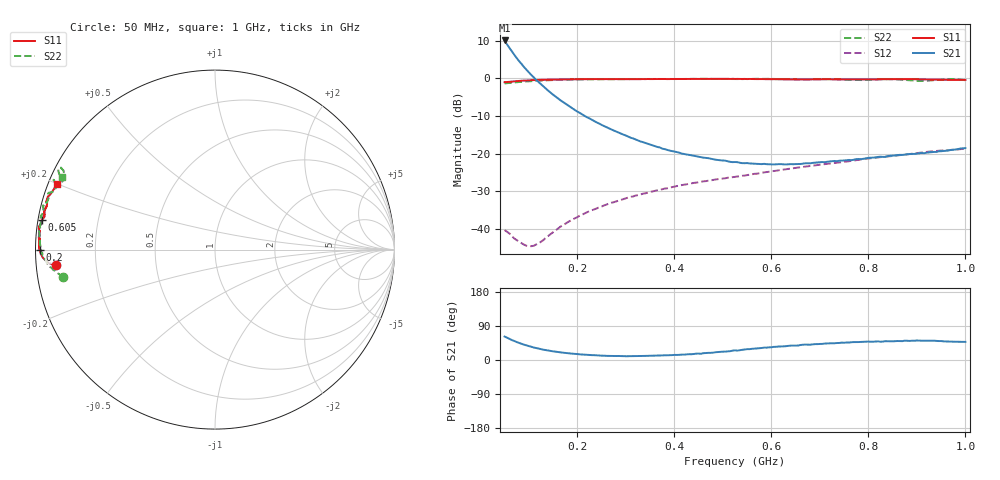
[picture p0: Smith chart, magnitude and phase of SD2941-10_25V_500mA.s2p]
!Agilent Technologies,E8358A,US42080673,A.04.86
!Agilent E8358A: A.04.86
!Date: Friday, June 09, 2006 14:44:03
!Correction: S11(Full 2 Port SOLT,1,2) S21(Full 2 Port SOLT,1,2) S12(Full 2 Port SOLT,1,2) S22(Full 2 Port SOLT,1,2)
!S2P File: Measurements: S11, S21, S12, S22:
# Hz S  MA  R 50
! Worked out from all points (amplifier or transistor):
!   191 points, 50 MHz to 1 GHz, reference 50 ohm
!   highest |S21| = 10.1 dB at 50 MHz (marker M1)
!   |S21| within 3 dB of that: start of sweep to 65.27 MHz
!   unconditionally stable (mu >= 1): 638.1 MHz to 683.3 MHz; 731.3 MHz to 825.9 MHz; 861.3 MHz to 965.3 MHz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
!   at 205 MHz: K = 0.28, MSG = 13.6 dB, |S12| = -36.4 dB
!   at 525 MHz: K = 0.64, MSG = 2.0 dB, |S12| = -26.1 dB
!   at 1 GHz: K = 1.14, MAG = -2.2 dB, |S12| = -18.6 dB
!   S11 on the Smith chart (normalised r, x): 50 MHz: 0.06, -0.05; 200 MHz: 0.01, -0.00; 605 MHz: 0.01, +0.08; 1 GHz: 0.02, +0.20
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5e7  0.8902 -174.5  3.194 61.9  0.009693 -4.6  0.858 -169.7
5.5e7  0.8963 -174.6  2.827 59.0  0.009186 -4.7  0.8649 -169.9
6.5e7  0.9078 -174.9  2.273 52.6  0.008091 -1.5  0.8774 -171.0
7.5e7  0.9195 -175.2  1.862 47.3  0.007109 2.7  0.8892 -171.7
9e7  0.9348 -175.7  1.417 40.5  0.006203 15.5  0.9079 -172.8
1e8  0.943 -176.2  1.205 36.5  0.005923 26.8  0.9159 -173.5
1.2e8  0.9554 -177.0  0.8951 29.9  0.006429 50.3  0.9329 -174.9
1.4e8  0.9641 -177.8  0.687 24.8  0.008084 63.8  0.9462 -176.4
1.65e8  0.9699 -178.7  0.5136 20.3  0.01075 72.1  0.9594 -178.0
2e8  0.9769 -179.9  0.3626 15.7  0.01437 77.4  0.9715 -179.8
2.1e8  0.9789 179.8  0.3324 14.6  0.01552 77.7  0.9724 179.7
2.7e8  0.9813 177.9  0.2098 10.7  0.02231 79.2  0.9775 177.0
3.7e8  0.9826 175.7  0.1212 11.7  0.03317 78.0  0.9817 172.9
4.15e8  0.9833 174.6  0.1006 14.2  0.0383 76.4  0.9836 171.0
5.25e8  0.9837 172.3  0.07757 25.3  0.04926 73.7  0.9791 167.6
6.05e8  0.9762 170.4  0.07207 34.7  0.05898 71.3  0.9841 165.3
6.85e8  0.9736 168.3  0.07553 41.0  0.06963 69.5  0.9743 162.0
7.9e8  0.9685 165.4  0.08565 48.0  0.08481 66.9  0.9515 158.4
8.45e8  0.9763 163.8  0.09413 49.4  0.09264 64.8  0.9797 156.7
8.95e8  0.9774 162.4  0.09946 50.8  0.101 63.0  0.9343 156.2
9.55e8  0.962 160.0  0.1088 49.2  0.1105 60.8  0.9703 151.9
1e9  0.9556 157.5  0.1188 47.9  0.1173 57.0  0.9454 154.6
